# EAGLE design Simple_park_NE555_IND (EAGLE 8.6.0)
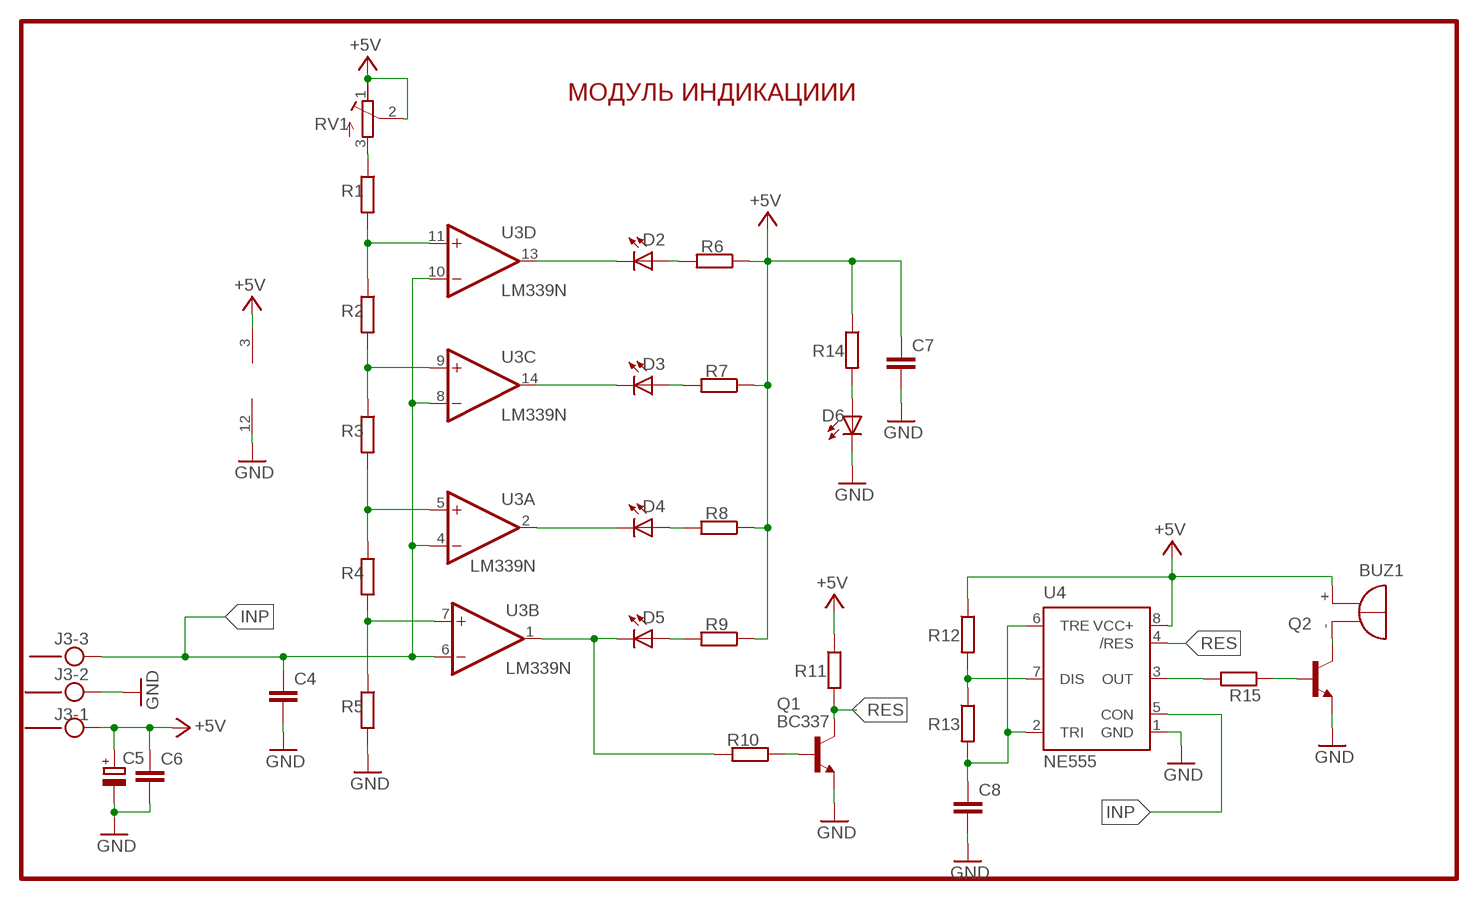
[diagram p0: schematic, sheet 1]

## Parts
BUZ1  F/HMB  [F/HMB]
C4  C-EUC1206  [C1206]
C5  CPOL-EUC/6032-28W  [C/6032-28W]
C6  C-EUC1206  [C1206]
C7  C-EUC1206  [C1206]
C8  C-EUC1206  [C1206]
D2  LED5MM  [LED5MM]
D3  LED5MM  [LED5MM]
D4  LED5MM  [LED5MM]
D5  LED5MM  [LED5MM]
D6  LED5MM  [LED5MM]
J3  MKDSN1,5/3-5,08  [MKDSN1,5/3-5,08]
Q1  BC337  [TO92]
Q2  BC33740T  BC337  [TO92]
R1  R-EU_R1206  [R1206]
R2  R-EU_R1206  [R1206]
R3  R-EU_R1206  [R1206]
R4  R-EU_R1206  [R1206]
R5  R-EU_R1206  [R1206]
R6  R-EU_R1206  [R1206]
R7  R-EU_R1206  [R1206]
R8  R-EU_R1206  [R1206]
R9  R-EU_R1206  [R1206]
R10  R-EU_R1206  [R1206]
R11  R-EU_R1206  [R1206]
R12  R-EU_R1206  [R1206]
R13  R-EU_R1206  [R1206]
R14  R-EU_R1206  [R1206]
R15  R-EU_R1206  [R1206]
RV1  R-TRIMM-3386-F  [R-TRIMM-3386F]
U3  LM339N  [DIL14]
U4  NE555  [DIL-08]

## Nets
+5V: BUZ1.+ C5.+ C6.1 C7.1 J3.1 R6.1 R7.1 R8.1 R9.1 R11.1 R12.1 R14.1 RV1.1(A) RV1.2(S) U3.3(P:V+) U4.8(VCC+)
GND: C4.2 C5.- C6.2 C7.2 C8.2 D6.K(C) J3.2 Q1.1(E) Q2.1(E) R5.2 U3.12(P:GND) U4.1(GND)
INP: C4.1 J3.3 U3.4(A:-IN) U3.6(B:-IN) U3.8(C:-IN) U3.10(D:-IN) U4.5(CON)
N$1: D4.K(C) U3.2(A:OUT)
N$4: C8.1 R13.2 U4.2(TRI) U4.6(TRE)
N$5: R12.2 R13.1 U4.7(DIS)
N$6: R1.2 R2.1 U3.11(D:+IN)
N$7: R2.2 R3.1 U3.9(C:+IN)
N$8: R3.2 R4.1 U3.5(A:+IN)
N$9: R4.2 R5.1 U3.7(B:+IN)
N$10: D2.K(C) U3.13(D:OUT)
N$11: D2.A R6.2
N$12: D3.K(C) U3.14(C:OUT)
N$13: D3.A R7.2
N$15: D4.A R8.2
N$16: D5.K(C) R10.2 U3.1(B:OUT)
N$17: D5.A R9.2
N$18: R1.1 RV1.3(E)
N$19: Q1.2(B) R10.1
N$21: Q2.2(B) R15.2
N$22: BUZ1.- Q2.3(C)
N$23: R15.1 U4.3(OUT)
N$24: D6.A R14.2
RES: Q1.3(C) R11.2 U4.4(/RES)

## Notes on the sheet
- МОДУЛЬ ИНДИКАЦИИИ

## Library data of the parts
BUZ1 = buzzer:F/HMB: BUZZER; OC_FARNELL: unknown; OC_NEWARK: unknown
C4 C6-C8 = rcl:C-EU: CAPACITOR, European symbol
C5 = rcl:CPOL-EU: POLARIZED CAPACITOR, European symbol
D2-D6 = led:LED: LED
J3 = con-phoenix-508:MKDSN1,5/3-5,08: MKDSN 1,5/ 3-5,08 Printklemme Nennstrom: 13,5 A Nennspannung: 250 V Rastermaß: 5,08 mm Polzahl: 3 Anschlussart: Schraubanschluss Montage: Löten Anschlussrichtung Leiter/Platine: 0 ° Artikelnummer: 1729131 Source: http://eshop.phoenixcontact.com .. 1729131.pdf
Q1 Q2 = transistor:BC337: NPN TRANSISTOR
R1-R15 = rcl:R-EU_: RESISTOR, European symbol
RV1 = rcl:R-TRIMM-3386-F
U3 = linear:LM339: Low Power Low Offset Voltage Quad Comparators with open collector; LM139/LM239/LM339/LM2901/LM3302
U4 = st-microelectronics:NE555: General purpose bipolar Timer; MF: Arrow Electronics; MPN: NE555N; OC_FARNELL: 1467742; OC_NEWARK: 89K1486

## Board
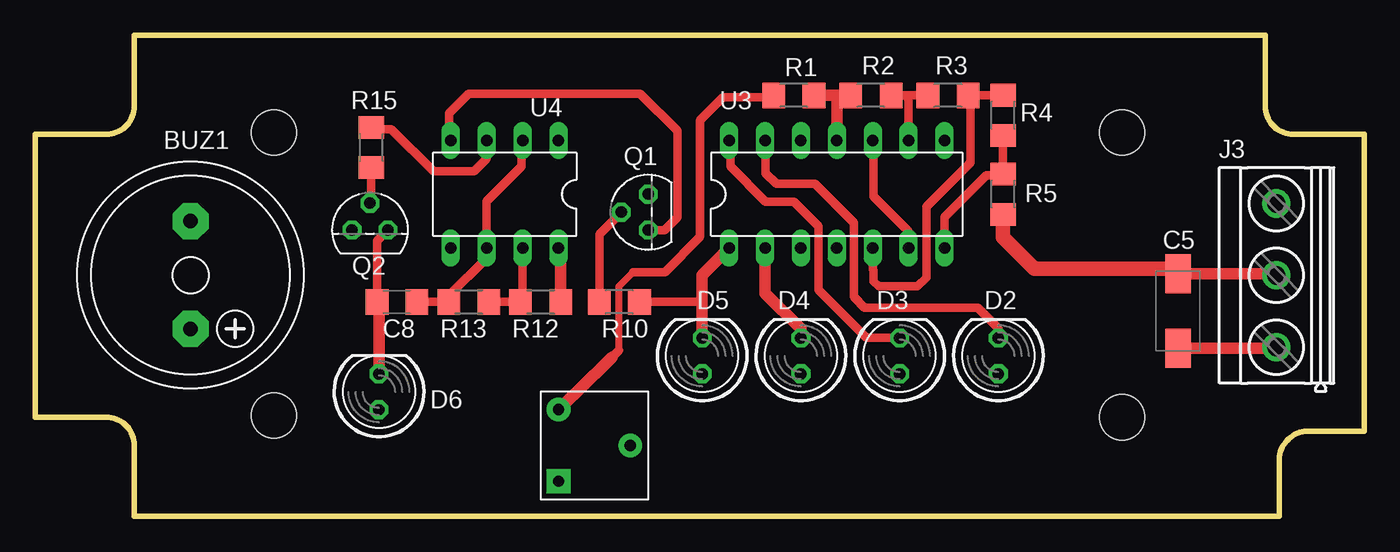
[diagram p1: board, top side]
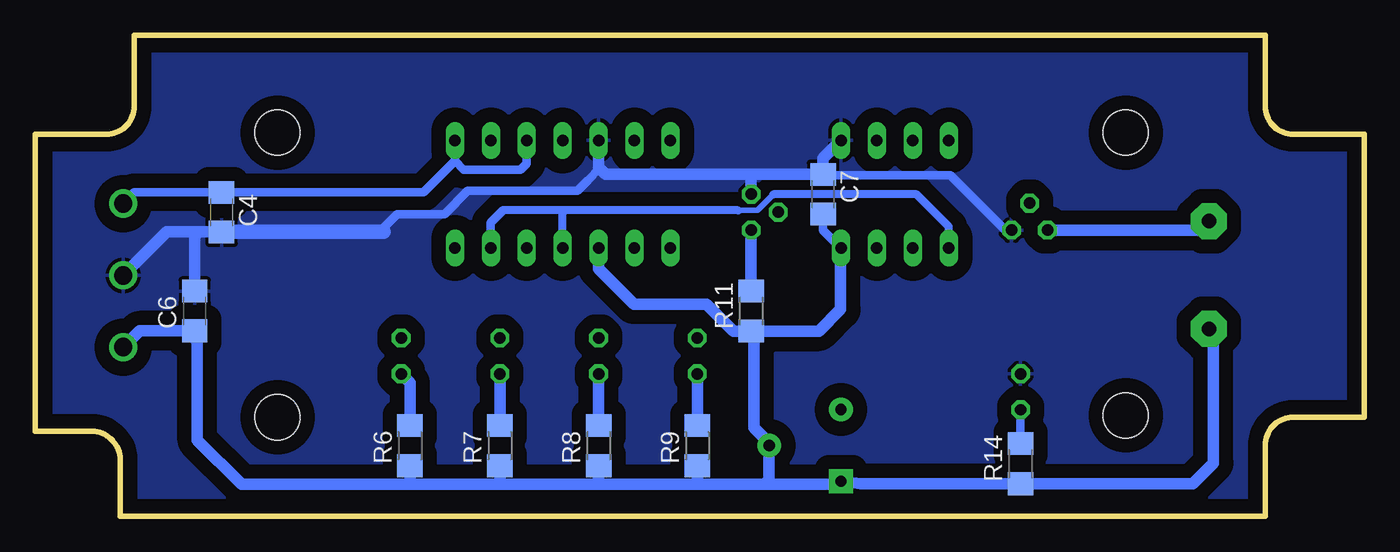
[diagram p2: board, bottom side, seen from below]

Size 94 x 34 mm. Coordinates in mm from the lower left corner, seen from the top.
Outline: 7,0 7,5 arc90 5,7 0,7 0,27 5,27 arc90 7,29 7,34 87,34 87,29 arc90 89,27 94,27 94,6 90,6 arc90 88,4 88,0 7,0
Copper layers (1*16): Top 0.035mm / dielectric 1.5mm / Bottom 0.035mm
Design rules "default": minimum track width 10mil, minimum drill 24mil, track to track 8mil, track to pad 8mil, pad to pad 8mil, via to via 8mil, smd to smd 8mil, copper to edge 40mil, drill to drill 8mil, minimum pad ring 10mil, minimum via ring 8mil, stop-mask expansion 4mil, vias tented up to drill 0mil, thermal gap 10mil
Holes 3.2 mm at 16.88,7.12 76.88,7 16.88,27.12 76.88,27.12

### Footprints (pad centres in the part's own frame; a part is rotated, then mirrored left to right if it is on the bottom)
F/HMB = drill 1.016 pad 2.54 octagon: + 3.81,0; - -3.81,0
C1206 = smd 1.6 x 1.8: 1 -1.4,0; 2 1.4,0
C/6032-28W = smd 2.75 x 1.8: + 2.625,0; - -2.625,0
LED5MM = drill 0.813 octagon: A -1.27,0; K 1.27,0
MKDSN1,5/3-5,08 = drill 1.3 pad 2: 1 -7.641,0.025; 2 -2.561,0.025; 3 2.519,0.025
TO92 = drill 0.813 octagon: 1 1.27,0; 2 0,1.905; 3 -1.27,0
R1206 = smd 1.6 x 1.803: 1 -1.422,0; 2 1.422,0
R-TRIMM-3386F = drill 0.8 pad 1.676 square: 1 0,0 | drill 0.8 pad 1.676: 2 5.08,2.54; 3 0,5.08
DIL14 = drill 0.813 long: 1 -7.62,-3.81; 2 -5.08,-3.81; 3 -2.54,-3.81; 4 0,-3.81; 5 2.54,-3.81; 6 5.08,-3.81; 7 7.62,-3.81; 8 7.62,3.81; 9 5.08,3.81; 10 2.54,3.81; 11 0,3.81; 12 -2.54,3.81; 13 -5.08,3.81; 14 -7.62,3.81
DIL-08 = drill 0.813 long: 1 -3.81,-3.81; 2 -1.27,-3.81; 3 1.27,-3.81; 4 3.81,-3.81; 5 3.81,3.81; 6 1.27,3.81; 7 -1.27,3.81; 8 -3.81,3.81

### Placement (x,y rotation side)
BUZ1  10.97,17.05 270 top
C4  80.83,21.5 270 bottom
C5  80.83,14.51 270 top
C6  82.73,14.51 90 bottom
C7  38.28,22.77 90 bottom
C8  25.58,15.14 180 top
D2  68.12,11.34 90 top
D3  61.14,11.34 90 top
D4  54.15,11.34 90 top
D5  47.17,11.34 90 top
D6  24.31,8.79 90 top
J3  87.81,19.59 90 top
Q1  43.36,21.5 90 top
Q2  23.68,20.23 0 top
R1  53.65,29.75 0 top
R2  59.11,29.75 0 top
R3  64.56,29.75 0 top
R4  68.44,28.34 270 top
R5  68.44,22.77 270 top
R6  67.49,4.99 90 bottom
R7  61.14,4.99 90 bottom
R8  54.15,4.99 90 bottom
R9  47.17,4.99 90 bottom
R10  41.32,15.14 0 top
R11  43.36,14.51 90 bottom
R12  35.74,15.14 180 top
R13  30.66,15.14 180 top
R14  24.31,3.71 90 bottom
R15  23.77,26.07 270 top
RV1  37.01,2.46 0 top
U3  56.69,22.77 0 top
U4  33.2,22.77 180 top

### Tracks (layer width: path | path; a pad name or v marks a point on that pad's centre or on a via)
+5V
  Top 0.813: C5.+ 87.72,11.88 J3.1 | R12.1 37.16,18.8 U4.8
  Bottom 0.61: C7.1 38.28,20.23 U4.8
  Bottom 0.813: C6.1 83.28,13.11 | 83.28,13.11 86.62,13.11 J3.1 | R11.1 44.62,13.09 46.53,15 51.66,15 54.16,17.5 U3.3 | R11.1 38.57,13.09 37.03,14.62 37.03,18.93 U4.8 | 83.28,13.11 82.53,12.36 82.53,5.38 79.41,2.25 67.66,2.25 | BUZ1.+ 10.66,12.93 10.66,3.75 12.12,2.29 R14.1 35.59,2.29 RV1.1 37.22,2.25 42.41,2.25 | 67.66,2.25 61.16,2.25 | 61.16,2.25 54.41,2.25 | 54.41,2.25 47.16,2.25 | 47.16,2.25 42.41,2.25 | 42.41,2.25 42.09,2.57 RV1.2 42.09,5.18 43.16,6.25 43.16,12.89 R11.1 | R9.1 47.17,2.26 47.16,2.25 | R8.1 54.15,2.5 54.41,2.25 | R7.1 61.14,2.27 61.16,2.25 | R6.1 67.49,2.42 67.66,2.25
GND
  Top 0.61: C8.2 24.18,19.46 Q2.1
  Top 0.813: C5.- 87.68,17.14 J3.2 | D6.K 24.31,15.02 C8.2
  Top 1.016: R5.2 68.44,19.71 70.66,17.5 80.46,17.5 C5.-
  Bottom 0.564: 54.91,23.75 54.07,24.59
  Bottom 0.61: 54.91,23.75 55.66,23 63.41,23 65.07,21.34 68.41,21.34 69.66,20.09 | Q2.1 25.39,20.23 29.29,24.12 38.24,24.12 C7.2
  Bottom 0.813: 43.36,24.16 C7.2 38.28,25.3 U4.1 | 43.36,24.16 53.65,24.16 54.07,24.59 54.15,24.67 U3.12 | Q1.1 43.36,24.16 | C4.2 82.41,20.09 | 82.41,20.09 84.72,20.09 J3.2 | C6.2 82.73,19.77 82.41,20.09
  Bottom 1.016: C4.2 69.66,20.09 69.37,20.09
  pour Bottom (isolate 1.016): -0.09,34 94.66,34 94.66,-0.25 -0.09,-0.25
INP
  Top 0.61: U3.6 61.77,20.14 59.28,22.62 59.28,26.52 U3.10
  Bottom 0.406: 41.78,22.75 42.91,21.62 44.28,21.62
  Bottom 0.564: U4.5 29.39,20.48 31.66,22.75 41.78,22.75 | 44.28,21.62 56.53,21.62 | 56.53,21.62 60.91,21.62 | U3.4 56.69,21.46 56.53,21.62
  Bottom 0.61: U3.10 59.23,24.93 59.66,24.5 63.69,24.5 64.31,25.12 | 64.31,25.12 U3.8 | J3.3 87,22.89 C4.1 66.55,22.89 64.31,25.12 | 60.91,21.62 61.78,20.75 61.78,18.96 U3.6
N$1
  Top 0.813: D4.K 54.15,13.24 51.61,15.78 U3.2
N$4
  Top 0.61: U4.2 34.41,26.52 34.41,24.75 31.93,22.27 U4.6 31.91,18.93 31.91,18.25 29.24,15.58 R13.2 C8.1
N$5
  Top 0.61: U4.7 34.47,15.3 R12.2 R13.1
N$6
  Top 0.813: R1.2 56.66,29.75 | 56.66,29.75 R2.1 | U3.11 56.69,29.71 56.66,29.75
N$7
  Top 0.61: R3.1 61.53,29.75 | 61.53,29.75 R2.2 | U3.9 61.77,29.51 61.53,29.75
N$8
  Top 0.61: U3.5 59.23,17.43 59.28,17.38 59.28,16.62 59.66,16.25 62.41,16.25 63.03,16.88 63.03,21.88 66.16,25 66.16,29.21 66.22,29.27 R3.2 66,29.77 R4.1
N$9
  Top 0.61: U3.7 64.31,21.16 67.28,24.12 68.38,24.12 R5.1 R4.2
N$10
  Top 0.61: D2.K 68.12,13.29 66.66,14.75 58.66,14.75 57.91,15.5 57.91,20.75 55.16,23.5 52.41,23.5 51.66,24.25 51.66,26.53 U3.13
N$11
  Bottom 0.813: R6.2 67.49,9.43 D2.A
N$12
  Top 0.61: D3.K 58.8,12.61 55.41,16 55.41,20.5 53.66,22.25 51.66,22.25 49.16,24.75 49.16,26.49 U3.14
N$13
  Bottom 0.813: R7.2 D3.A
N$15
  Bottom 0.813: R8.2 D4.A
N$16
  Top 0.61: R10.2 47.06,15.14 47.17,15.25
  Top 0.813: D5.K 47.17,15.25 47.17,17.05 U3.1
N$17
  Bottom 0.813: R9.2 D5.A
N$18
  Top 0.5: 41.28,11.75 41.28,16.25 42.28,17.25
  Top 0.61: 40.78,11.25 41.28,11.75 | 42.28,17.25 44.53,17.25 47.03,19.75 47.03,28 48.66,29.62 52.11,29.62 R1.1
  Top 0.813: RV1.3 38.33,8.79 40.78,11.25
N$19
  Top 0.61: R10.1 39.9,19.94 Q1.2
N$21
  Top 0.61: R15.2 23.77,22.23 Q2.2
N$22
  Bottom 0.813: Q2.3 11.61,20.23 BUZ1.-
N$23
  Top 0.61: U4.3 31.93,25.27 31.04,24.38 28.16,24.38 25.16,27.38 23.88,27.38 R15.1
N$24
  Bottom 0.61: R14.2 D6.A
RES
  Top 0.61: Q1.3 44.51,20.23 45.41,21.12 45.41,27.25 42.78,29.88 30.66,29.88 29.29,28.5 29.29,26.68 U4.4
  Bottom 0.813: Q1.3 R11.2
